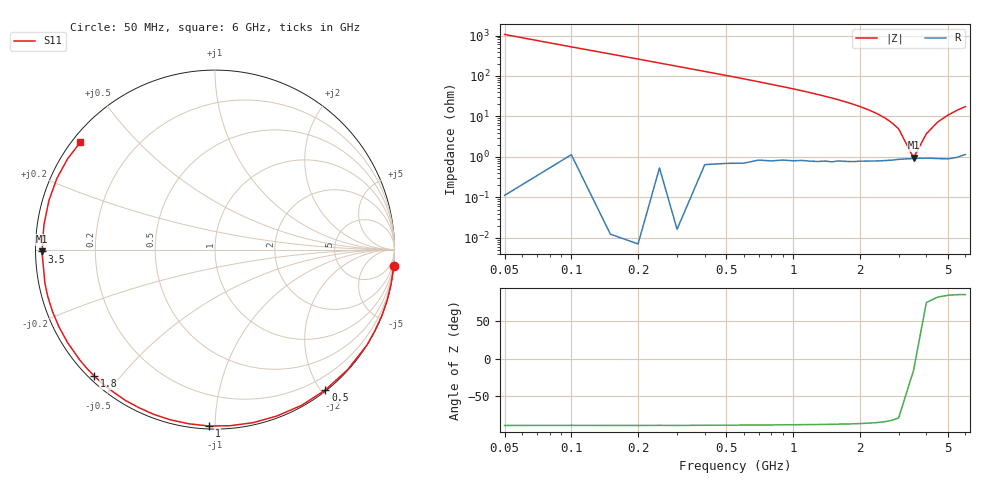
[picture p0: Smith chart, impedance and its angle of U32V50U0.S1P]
! SIEMENS Discrete & RF Semiconductors
! BBY53-02W
! Si Tuning Diode in SCD-80
! VR = 2.5 V
! S-Parameters:  September  1997
# GHz  S  MA  R  50
!  f  S11
! GHz  MAG  ANG
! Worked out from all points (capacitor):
!   34 points, 50 MHz to 6 GHz, reference 50 ohm
!   read as one part to ground: C = 3.03 pF near 50 MHz
!   lowest |Z| = 954 mohm at 3.5 GHz (marker M1)
!   series resonance near 3.534 GHz, so ESL is about 670 pH
!   S11 on the Smith chart (normalised r, x): 50 MHz: 0, -21; 500 MHz: 0.01, -2.06; 1 GHz: 0.02, -0.97; 1.8 GHz: 0.02, -0.43; 3.5 GHz: 0.02, -0.01; 6 GHz: 0.02, +0.35
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0.05  1 -5.4
0.15  1 -16.3
0.25  0.9988 -26.9
0.3  1 -32.1
0.4  0.9967 -42.2
0.5  0.9947 -51.8
0.6  0.9928 -60.9
0.7  0.9892 -69.5
0.8  0.9875 -77.6
0.9  0.9847 -85.2
1  0.9835 -92.0
1.1  0.9813 -98.6
1.3  0.9793 -110.4
1.5  0.9774 -120.6
1.6  0.9751 -125.2
1.8  0.9742 -133.6
2  0.9724 -141.0
2.2  0.9712 -147.7
2.4  0.9702 -153.7
2.6  0.9689 -159.2
2.8  0.9677 -164.3
3  0.966 -168.9
3.5  0.964 -179.4
4  0.9633 171.7
4.5  0.9648 163.5
5  0.9663 155.7
5.5  0.9644 148.3
6  0.9597 141.4
